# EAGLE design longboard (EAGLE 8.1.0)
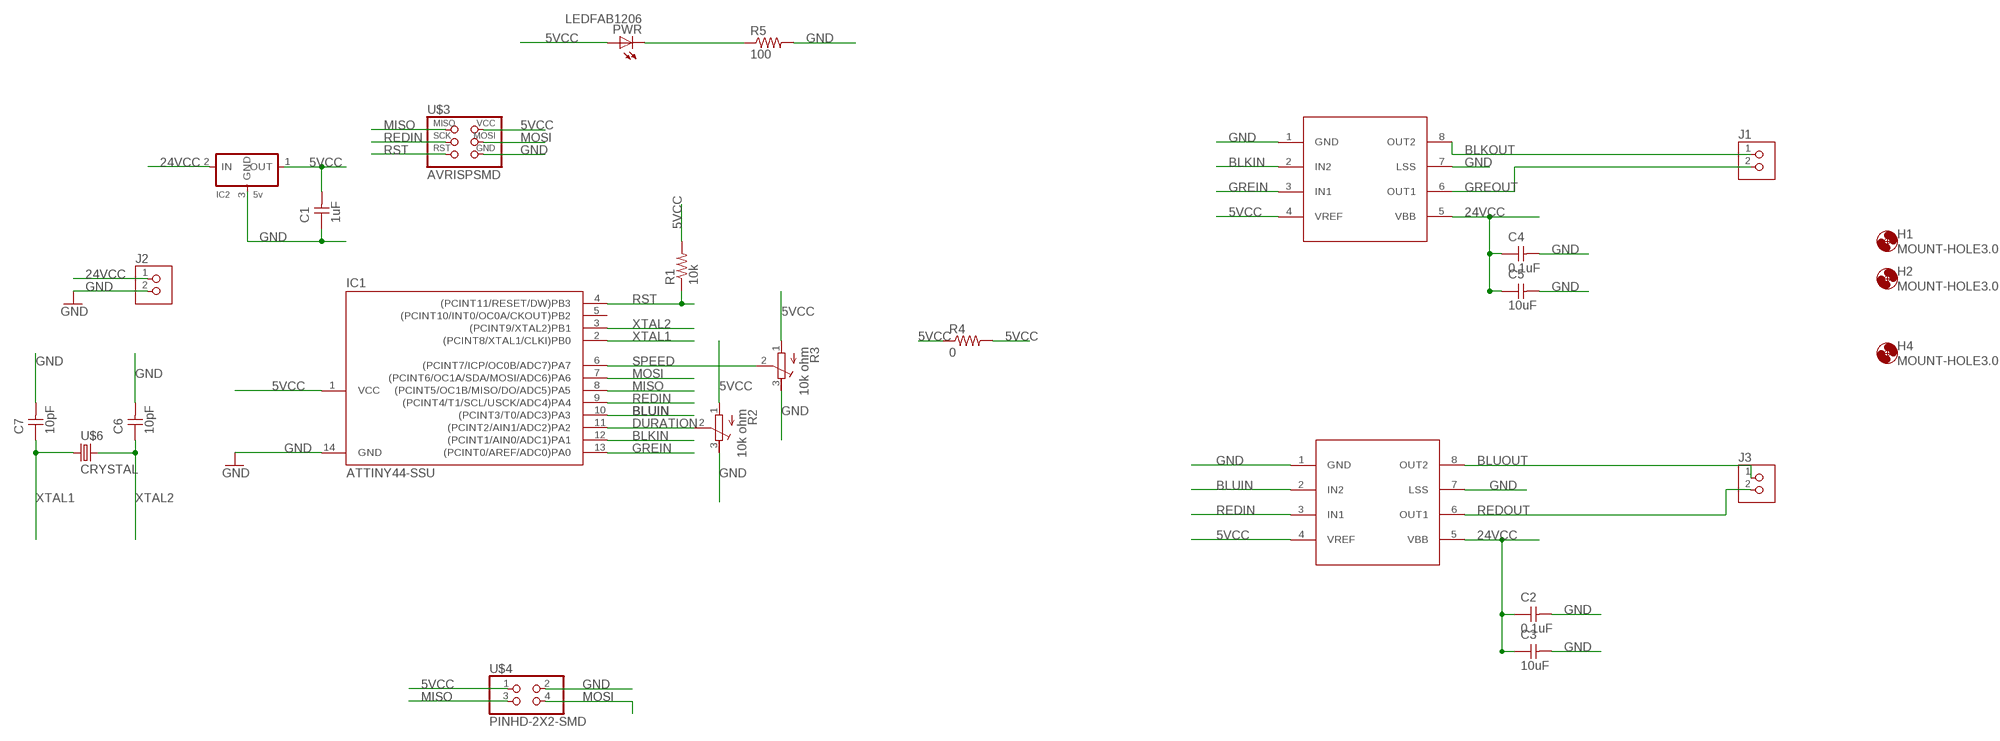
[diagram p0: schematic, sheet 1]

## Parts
C1  1uF  CAP-UNPOLARIZEDFAB  [C1206FAB]
C2  0.1uF  CAP-UNPOLARIZEDFAB  [C1206FAB]
C3  10uF  CAP-UNPOLARIZEDFAB  [C1206FAB]
C4  0.1uF  CAP-UNPOLARIZEDFAB  [C1206FAB]
C5  10uF  CAP-UNPOLARIZEDFAB  [C1206FAB]
C6  10pF  CAP-UNPOLARIZEDFAB  [C1206FAB]
C7  10pF  CAP-UNPOLARIZEDFAB  [C1206FAB]
H1  MOUNT-HOLE3.0  [3,0]
H2  MOUNT-HOLE3.0  [3,0]
H4  MOUNT-HOLE3.0  [3,0]
IC1  ATTINY44-SSU  [SOIC14]
IC2  5v  REGULATORSOT23  [SOT23]
J1  TERM-1X02-FABLAB  [ED555DS-2DS]
J2  TERM-1X02-FABLAB  [ED555DS-2DS]
J3  TERM-1X02-FABLAB  [ED555DS-2DS]
PWR  LEDFAB1206  [LED1206FAB]
R1  10k  RES-US1206FAB  [R1206FAB]
R2  10k ohm  R-TRIMM3103  [RTRIM3103]
R3  10k ohm  R-TRIMM3103  [RTRIM3103]
R4  0  RES-US1206FAB  [R1206FAB]
R5  100  RES-US1206FAB  [R1206FAB]
U$1  A4953-H-BRIDGE-MOTOR-DRIVER  [SOIC8]
U$2  A4953-H-BRIDGE-MOTOR-DRIVER  [SOIC8]
U$3  AVRISPSMD  [2X03SMD]
U$4  PINHD-2X2-SMD  [2X02SMD]
U$6  CRYSTAL  [2-SMD-5X3MM]

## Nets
5VCC: C1.2 IC1.1(VCC) IC2.1(OUT) PWR.1(A) R1.2 R2.1(A) R3.1(A) R4.1 R4.2 U$1.4(VREF) U$2.4(VREF) U$3.2(VCC) U$4.1
24VCC: C2.1 C3.1 C4.1 C5.1 IC2.2(IN) J2.1 U$1.5(VBB) U$2.5(VBB)
BLKIN: IC1.12((PCINT1/AIN0/ADC1)PA1) U$1.2(IN2)
BLKOUT: J1.1 U$1.8(OUT2)
BLUIN: IC1.10((PCINT3/T0/ADC3)PA3) U$2.2(IN2)
BLUOUT: J3.1 U$2.8(OUT2)
DURATION: IC1.11((PCINT2/AIN1/ADC2)PA2) R2.2(S)
GND: C1.1 C2.2 C3.2 C4.2 C5.2 C6.2 C7.2 IC1.14(GND) IC2.3(GND) J2.2 R2.3(E) R3.3(E) R5.2 U$1.1(GND) U$1.7(LSS) U$2.1(GND) U$2.7(LSS) U$3.6(GND) U$4.2
GREIN: IC1.13((PCINT0/AREF/ADC0)PA0) U$1.3(IN1)
GREOUT: J1.2 U$1.6(OUT1)
MISO: IC1.8((PCINT5/OC1B/MISO/DO/ADC5)PA5) U$3.1(MISO) U$4.3
MOSI: IC1.7((PCINT6/OC1A/SDA/MOSI/ADC6)PA6) U$3.4(MOSI) U$4.4
N$6: PWR.2(C) R5.1
REDIN: IC1.9((PCINT4/T1/SCL/USCK/ADC4)PA4) U$2.3(IN1) U$3.3(SCK)
REDOUT: J3.2 U$2.6(OUT1)
RST: IC1.4((PCINT11/RESET/DW)PB3) R1.1 U$3.5(RST)
SPEED: IC1.6((PCINT7/ICP/OC0B/ADC7)PA7) R3.2(S)
XTAL1: C7.1 IC1.2((PCINT8/XTAL1/CLKI)PB0) U$6.P$1
XTAL2: C6.1 IC1.3((PCINT9/XTAL2)PB1) U$6.P$2
Unconnected: IC1.5((PCINT10/INT0/OC0A/CKOUT)PB2)

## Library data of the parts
C1-C7 = fab:CAP-UNPOLARIZED
H1 H2 H4 = holes:MOUNT-HOLE: MOUNTING HOLE with drill center marker
IC1 = fab:ATTINY44
IC2 = fab:REGULATOR
J1-J3 = fab:TERM-1X02: 3.5mm terminal block, 2 positions ED555-2DS as found in the fablab inventory.
PWR = fab:LED: LED
R1 R4 R5 = fab:RES-US: Resistor (US Symbol)
R2 R3 = resistor:R-TRIMM: Trimm resistor
U$1 U$2 = fab:A4953-H-BRIDGE-MOTOR-DRIVER
U$3 = fab:AVRISP
U$4 = fab:PINHD-2X2-SMD
U$6 = fab:CRYSTAL

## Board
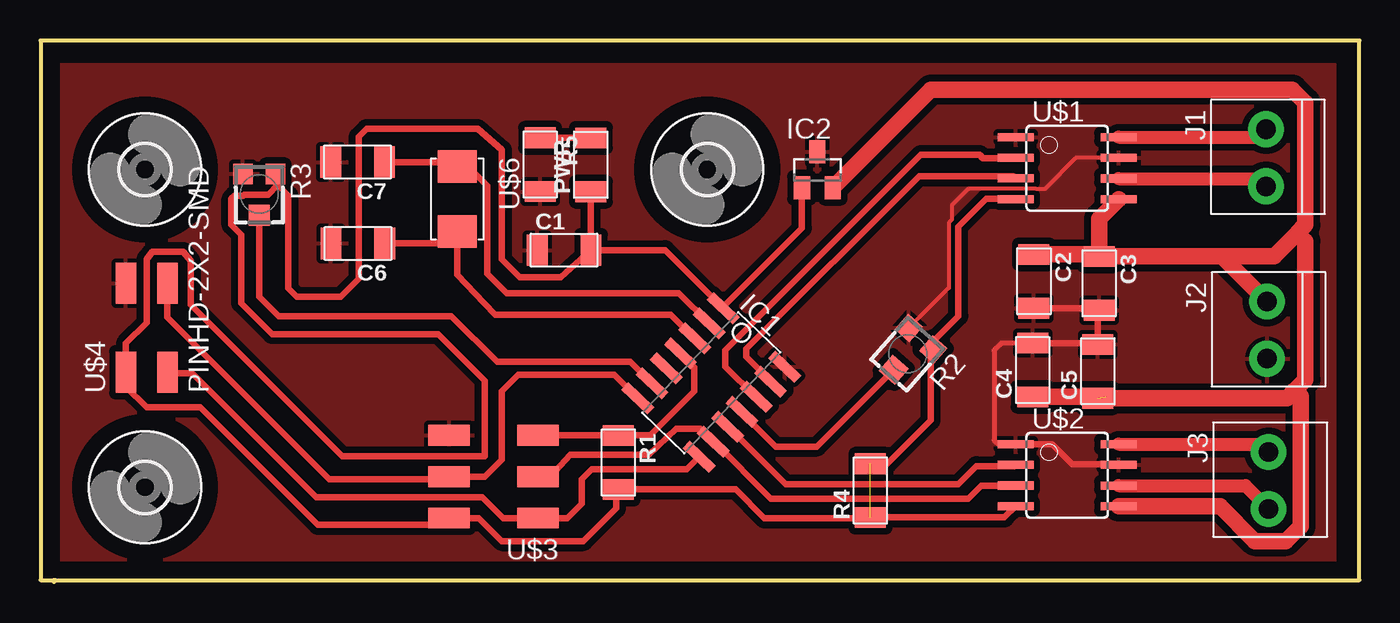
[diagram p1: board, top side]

Size 80.9 x 33.2 mm. Coordinates in mm from the lower left corner, seen from the top.
Outline: 0.9,0.1 80.9,0.1 80.9,33.2 0,33.2 0,0.1 0.8,0.1 0.8,0
Copper layers (1*16): Top 0.035mm / dielectric 1.5mm / Bottom 0.035mm
Design rules "FabLabOulu_DRC *": minimum track width 16mil, minimum drill 24mil, track to track 0.25mm, track to pad 0.25mm, pad to pad 0.25mm, via to via 0.25mm, smd to smd 0.25mm, copper to edge 40mil, drill to drill 8mil, minimum pad ring 10mil, minimum via ring 8mil, stop-mask expansion 4mil, vias tented up to drill 0mil, thermal gap 10mil

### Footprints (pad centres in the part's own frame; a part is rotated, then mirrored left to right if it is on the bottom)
C1206FAB = smd 1.27 x 1.905: 1 -1.651,0; 2 1.651,0
3,0 = hole 3: 0,0
SOIC14 = smd 0.61 x 2.21: 1 -3.81,-2.603; 2 -2.54,-2.603; 3 -1.27,-2.603; 4 0,-2.603; 5 1.27,-2.603; 6 2.54,-2.603; 7 3.81,-2.603; 8 3.81,2.603; 9 2.54,2.603; 10 1.27,2.603; 11 0,2.603; 12 -1.27,2.603; 13 -2.54,2.603; 14 -3.81,2.603
SOT23 = smd 1 x 1.4: 1 -0.95,-1.1; 2 0.95,-1.1; 3 0,1.1
ED555DS-2DS = drill 1.2 pad 2.184: 1 1.8,0; 2 -1.7,0
LED1206FAB = smd 1.27 x 1.905: 1 -1.651,0; 2 1.651,0
R1206FAB = smd 1.27 x 1.905: 1 -1.651,0; 2 1.651,0
RTRIM3103 = smd 1.2 x 1.25: 1 -1,-1.225; 3 1,-1.225 | smd 1.3 x 1.3: 2 0,1.3
SOIC8 = smd 0.5 x 2.2: 1 -1.905,-3.154; 2 -0.645,-3.154; 3 0.625,-3.154; 4 1.895,-3.154; 5 1.905,3.154; 6 0.635,3.154; 7 -0.635,3.154; 8 -1.905,3.154
2X03SMD = smd 2.54 x 1.27: 1 -2.54,2.54; 2 2.92,2.54; 3 -2.54,0; 4 2.92,0; 5 -2.54,-2.54; 6 2.92,-2.54
2X02SMD = smd 2.54 x 1.27: 1 -2.54,1.27; 2 2.92,1.27; 3 -2.54,-1.27; 4 2.92,-1.27
2-SMD-5X3MM = smd 2 x 2.4: P$1 -2,0; P$2 2,0

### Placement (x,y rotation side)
C1  32.11,20.35 0 top
C2  60.94,18.44 270 top
C3  64.94,18.32 270 top
C4  60.86,13 90 top
C5  64.86,12.92 90 top
C6  19.46,20.76 180 top
C7  19.44,25.76 180 top
H1  6.4,5.8 0 top
H2  6.4,25.3 0 top
H4  40.9,25.3 0 top
IC1  41.14,12.22 226.4 top
IC2  47.65,25.28 0 top
J1  75.19,25.97 90 top
J2  75.24,15.39 90 top
J3  75.34,6.17 90 top
PWR  33.75,25.59 90 top
R1  35.44,7.32 270 top
R2  53.2,14 138.6 top
R3  13.4,23.8 180 top
R4  50.9,5.6 90 top
R5  30.64,25.6 270 top
U$1  62.98,25.38 270 top
U$2  62.98,6.54 270 top
U$3  27.97,6.45 180 top
U$4  6.5,15.4 90 top
U$6  25.56,23.49 270 top

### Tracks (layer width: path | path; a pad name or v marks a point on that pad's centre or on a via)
5VCC  (1 unrouted)
  Top 0.406: C1.2 33.76,23.93 PWR.1 33.91,24.1 | IC2.1 46.7,21.7 41.88,16.88 IC1.1 38.31,20.35 C1.2 | U$2.4 59.13,3.95 R4.1 50.85,3.9 44.4,3.9 42.63,5.67 R1.2 35.3,5.53 35.3,4.5 33.3,2.5 28.3,2.5 26.89,3.91 U$3.2 24.64,3.5 17,3.5 9.8,10.7 6.5,10.7 5.23,11.97 U$4.1 5.23,14.63 6.5,15.9 6.5,19.8 6.85,20.25 8.75,20.25 9.2,19.7 9.2,17 18.5,7.7 27.25,7.7 27.25,12.35 24.4,15.2 14.2,15.2 12.3,17.1 12.3,21.3 11.7,21.9 11.7,23.5 11.9,23.7 12.44,23.7 12.5,23.76 13.96,23.76 14.55,24.35 | R4.2 51.95,7.25 54.6,9.9 54.6,14.1 R2.1 54.76,14.76 56.3,16.3 56.3,21.8 58,23.5 59.81,23.5 U$1.4 | R3.1 14.4,24.5 14.55,24.35 | 14.55,24.35 15.2,23.7 15.2,18 15.7,17.5 18.4,17.5 19.5,18.6 19.5,27.3 20,27.8 26.8,27.8 28.3,26.5 28.3,19.8 29.4,18.7 31.91,18.7 C1.2
24VCC  (1 unrouted)
  Top 1.016: C2.1 64.82,20.09 C3.1 | C4.1 65.35,11.35 65.4,11.3 | C3.1 72.46,19.97 | J2.1 72.46,19.97 | 72.46,19.97 75.67,19.97 77.1,21.4 | 77.1,21.4 77.6,21.9 77.6,29.4 76.8,30.2 54.62,30.2 IC2.2 | C3.1 64.94,22.28 U$1.5 | C5.1 76.47,11.27 76.95,11.75 | 76.95,11.75 77.6,12.4 77.6,20.9 77.1,21.4 | U$2.5 72.37,4.63 74.5,2.5 76.4,2.5 77.3,3.4 77.3,11.4 76.95,11.75
BLKIN
  Top 0.406: IC1.12 43.86,11.34 42,13.2 42,14.2 54,26.2 57.6,26.2 57.8,26 59.8,26 U$1.2
BLKOUT
  Top 0.813: U$1.8 74.71,27.29 J1.1
BLUIN
  Top 0.406: IC1.10 42.2,9.51 45.7,6 56.3,6 57.4,7.1 59.74,7.1 U$2.2
BLUOUT
  Top 0.813: U$2.8 74.87,8.45 J3.1
DURATION
  Top 0.406: IC1.11 43.02,10.38 45.1,8.3 47.62,8.3 R2.2
GND
  Top 0.254: U$1.7 63.52,26.02 61.6,24.1 61.09,24.1 61.08,24.11 56.91,24.11 55.9,23.1 55.9,22.22 55.72,22.04 55.72,18.04 R2.3
  Top 0.305: C4.2 58.95,14.65 58.5,14.2 58.5,8.7 58.8,8.4 59.78,8.4 U$2.1
  Top 0.406: U$2.1 62.05,8.45 63.3,7.2 66.11,7.2 U$2.7 | C4.2 64.78,14.65 C5.2 64.86,16.59 C3.2 64.82,16.79 C2.2
  pour Top (isolate 0.406): 1,0.1 79.4,0.1 79.4,31.7 1,31.7
GREIN
  Top 0.406: IC1.13 44.78,12.32 43.3,13.8 43.3,14.3 53.9,24.9 59.68,24.9 U$1.3
GREOUT
  Top 0.813: U$1.6 74.72,24.75 J1.2
MISO
  Top 0.406: U$4.3 7.83,12.8 9.3,12.8 16.9,5.2 27.1,5.2 28.39,3.91 U$3.1 32.31,3.91 33.2,4.8 33.2,6.3 33.8,6.9 39.63,6.9 IC1.8
MOSI
  Top 0.406: U$4.4 7.77,16.23 17.7,6.3 24.9,6.3 U$3.4 27.25,6.45 28.3,7.5 28.3,11.7 29.3,12.7 35.18,12.7 IC1.7
N$6
  Top 0.406: R5.1 33.74,27.25 PWR.2
REDIN
  Top 0.406: U$2.3 59.81,5.9 57.7,5.9 56.9,5.1 44.8,5.1 41.31,8.59 IC1.9 40.46,9.4 39,9.4 37.3,7.8 32.5,7.8 31.25,6.45 U$3.3
REDOUT
  Top 0.813: U$2.6 73.91,5.91 J3.2
RST
  Top 0.406: 35.3,8.99 U$3.5 | 35.3,8.99 37.39,8.99 40.1,11.7 40.1,13.17 IC1.4 | R1.1 35.32,8.97 35.3,8.99
SPEED
  Top 0.406: R3.2 13.4,17.5 14.6,16.3 25.2,16.3 28,13.5 36.18,13.5 IC1.6
XTAL1
  Top 0.406: C7.1 25.29,25.76 U$6.P$1 26.21,25.49 27.4,24.3 27.4,18.9 28.6,17.7 39.16,17.7 IC1.2
XTAL2
  Top 0.406: C6.1 24.83,20.76 U$6.P$2 25.56,18.84 27.2,17.1 27.9,16.4 38.67,16.4 IC1.3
